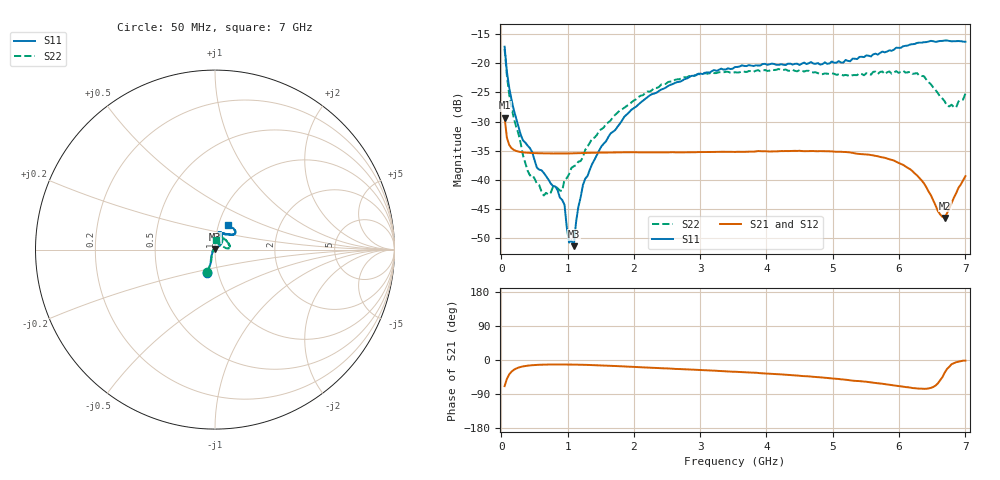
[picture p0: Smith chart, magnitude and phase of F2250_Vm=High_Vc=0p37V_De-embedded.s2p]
! Integrated Device Technology
! Corporate Headquarters
! 6024 Silver Creek Valley Road
! San Jose, CA 95138  USA
! Phone:  1-408-284-8200
! Toll Free:  1-800-223-1366
! Webpage:  http://www.idt.com/
! Timing and RF Division
! 515 Groton Road, Suite 102
! Westford, MA 01886-6024
! Device:  F2250
! Description: Voltage Variable RF Attenuator
! Frequency:  50.0 -  6000.00 MHz
! Package:  3x3 mm Thin QFN Plastic Package: 16 pin
! Ports:  2 RF, 3 DC
!  Pin  1  = GND
!  Pin  2  = NC
!  Pin  3  = RF1  = Port 1
!  Pin  4  = NC
!  Pin  5  = GND
!  Pin  6  = GND
!  Pin  7  = GND
!  Pin  8  = GND
!  Pin  9  = NC
!  Pin 10  = RF2  = Port 2
!  Pin 11  = NC
!  Pin 12  = GND
!  Pin 13  = GND
!  Pin 14  = VCNTRL
!  Pin 15  = VDD
!  Pin 16  = VMODE
! Vcntrl:  0.370 Volts
! Vmode:  +3.300 Volts
! Vdd:  +3.30  Volts
! Current:  1.259 mA
! Data:  The device was measured on a the F2250 evaluation board which has
!  individual transmission lines to the RF pins.  Data was collected
!  using a calibrated network analyzer.  The evaluation board was
!  de-embedded using a TRL calibration technique.
!  The reference plane is the edge of the package pin.
! Misc:  SN 10
!  Action Tracker AT0258
! Date Measured:  2014-11-26
! Date:  2015-10-15  MJV
! Note:
!  Integrated Device Technology supplies this data as a sample of measured
!  data at the package pin for this product.  Your particular data for this
!  product may vary.
!  Data was taken at 25 degrees C.
!  Integrated Device Technology reserves the right to change this data at anytime.
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# GHz S dB R 50
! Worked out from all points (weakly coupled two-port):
!   201 points, 50 MHz to 7 GHz, reference 50 ohm
!   highest |S21| = -29.34 dB at 50 MHz (marker M1); lowest = -46.5 dB at 6.687 GHz (marker M2)
!   lowest |S11| = -51.3 dB at 1.093 GHz (marker M3), VSWR 1.01, Z = 50 + j0.271 ohm
!   |S11| at or under -10 dB: start of sweep to end of sweep
!   |S22| runs from -42.7 to -17.6 dB; largest |S21 - S12| = 6.4e-05
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0.05  -17.17 -108.5  -29.34 -68.9  -29.33 -68.9  -17.56 -109.6
0.08475  -21.47 -107.4  -32.77 -49.6  -32.76 -49.6  -22.14 -106.8
0.189  -28.00 -120.0  -34.85 -25.9  -34.85 -25.9  -29.43 -119.2
0.328  -33.23 -134.0  -35.26 -16.9  -35.27 -16.9  -35.81 -132.3
0.43225  -34.54 -145.3  -35.36 -14.2  -35.36 -14.2  -39.23 -161.3
0.5365  -37.88 -154.7  -35.41 -12.9  -35.41 -12.9  -40.65 -176.8
0.64075  -38.78 -162.6  -35.44 -12.2  -35.44 -12.2  -42.66 154.9
0.91875  -43.42 156.0  -35.46 -11.9  -35.46 -11.9  -41.87 109.6
0.9535  -44.24 170.5  -35.46 -11.9  -35.46 -11.9  -39.92 108.8
1.023  -50.73 140.3  -35.45 -12.0  -35.45 -12.0  -38.99 90.6
1.0925  -51.34 89.3  -35.43 -12.1  -35.43 -12.1  -37.66 82.4
1.162  -44.62 56.0  -35.42 -12.3  -35.42 -12.4  -36.85 71.0
1.2315  -40.85 40.5  -35.39 -12.6  -35.39 -12.6  -36.07 62.4
1.6485  -32.02 41.2  -35.30 -15.3  -35.30 -15.4  -29.82 52.7
2.37825  -24.75 46.6  -35.27 -21.3  -35.27 -21.3  -24.07 50.2
3.525  -20.65 71.7  -35.20 -31.0  -35.19 -31.0  -21.55 71.1
4.7065  -20.06 72.0  -35.04 -44.3  -35.04 -44.4  -21.58 69.2
5.85325  -17.79 40.5  -36.45 -65.2  -36.45 -65.3  -21.39 21.6
6.3745  -16.40 41.0  -40.57 -76.1  -40.59 -76.2  -22.21 5.4
6.68725  -16.11 47.9  -46.49 -33.6  -46.50 -33.3  -26.53 27.0
6.861  -16.22 54.5  -42.26 -5.8  -42.22 -5.9  -27.56 57.8
7  -16.32 62.4  -39.35 -1.7  -39.31 -1.9  -25.19 85.2
